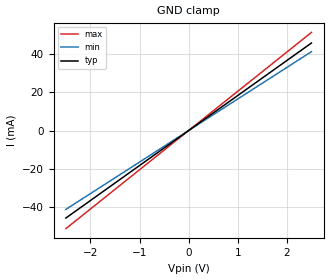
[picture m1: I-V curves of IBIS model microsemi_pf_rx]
|   Microsemi MPF300XT IBIS-AMI Model
[IBIS Ver]   6.0
[Disclaimer] THIS IBIS MODEL HAS BEEN CREATED BY THE SIGNAL
   INTEGRITY SOFTWARE SPICE WRAPPING PROCESS.
   THESE IBIS MODELS AREPROVIDED "AS IS" WITH NO
   WARRANTY WHATSOEVER AND SIGNAL INTEGRITY SOFTWARE
   SPECIFICALLY DISCLAIMS ANY IMPLIED WARRANTIES OF
   MERCHANTABILITY, FITNESS FOR A PARTICULAR PURPOSE,
   OR AGAINST INFRINGEMENT.
[File Name]  mpf300xt_rx_ami.ibs
[Date]   Feb 29, 2018
[File Rev]   1.0
[Source]   Microsemi PolarFire MPF300XT AMI model provided by SiSoft
[Notes]   Revision 1.0
|   Initial Release
|   DFE settings are not supported
[Copyright]  Copyright 2018, Microsemi Corporation, All Rights Reserved.
|   COMPONENT: microsemi_pf_serdes
[Component] microsemi_pf_serdes
[Manufacturer]  Microsemi
[Package]
R_pkg   0.001m  NA NA
L_pkg   0.000nH NA NA
C_pkg   0.000pF NA NA
[Pin] signal_name   model_name   R_pin L_pin C_pin
1   microsemi_pf_rx_p   microsemi_pf_rx   NA   NA   NA
2   microsemi_pf_rx_n   microsemi_pf_rx   NA   NA   NA
[Diff Pin] inv_pin  vdiff tdelay_typ tdelay_min tdelay_max
1   2   0.050 na   na   na
| Models and submodels in the file (1): microsemi_pf_rx (Input)
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|   MODEL: microsemi_pf_rx
[Model]   microsemi_pf_rx
|SiSoft ModelSignature3 115b805d4d8838d44e017cc8bd906e146d2f2c0c2739a659b70f08e399bdd595 Certified
Model_type Input
Vinl = .05
Vinh = .05
|   typ   min   max
C_comp   0.7pF 0.7pF 0.7pF
[Model Spec]
[Algorithmic Model]
Executable Linux_gcc4.4.7_64   microsemi_PF_rx_glnxa64.so microsemi_pf_rx.ami
Executable Windows_VisualStudio7.1.3088_64  microsemi_PF_rx_win64.dll  microsemi_pf_rx.ami
[End Algorithmic Model]
[Temperature Range]  65   125  -40
[Voltage Range]   1.0  1.0  1.0
[GND Clamp]
-2.5V     -45.5mA    -41mA      -51mA
0V        0A         0A         0A
2.5V      45.5mA     41mA       51mA
